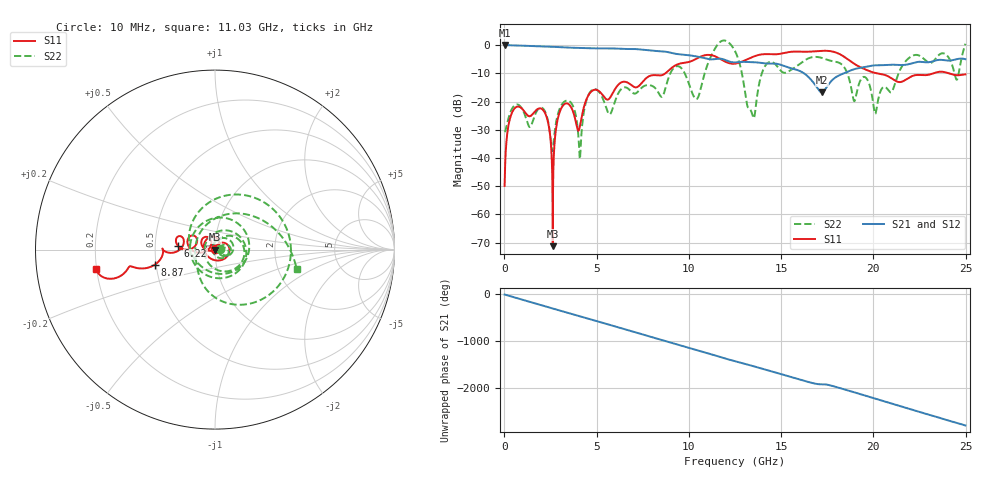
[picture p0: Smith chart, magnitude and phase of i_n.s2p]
!Keysight Technologies,N5245B,MY57181346,A.12.70.07
!Automatic Fixture Removal (AFR)
!Date: Wednesday, November 07, 2018 11:53:51 AM
!S2P File: Measurements: S11,S21,S12,S22:
# MHz S  RI  R 50
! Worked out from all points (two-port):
!   2499 points, 10 MHz to 24.99 GHz, reference 50 ohm
!   highest |S21| = 0.00 dB at 10 MHz (marker M1); lowest = -16.8 dB at 17.21 GHz (marker M2)
!   |S21| within 3 dB of the highest: start of sweep to 9.215 GHz
!   lowest |S11| = -71.3 dB at 2.62 GHz (marker M3), VSWR 1.00, Z = 50 - j0.0251 ohm
!   |S11| at or under -10 dB: start of sweep to 8.728 GHz; 20.19 GHz to 23.26 GHz (3.073 GHz wide, 14.1 % of centre); 24.08 GHz to end of sweep
!   |S22| runs from -40.4 to 1.6 dB; largest |S21 - S12| = 1.4e-15
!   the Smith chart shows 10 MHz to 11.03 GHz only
!   S11 on the Smith chart (normalised r, x): 10 MHz: 1.01, +0.00; 6.22 GHz: 0.66, +0.03; 8.87 GHz: 0.49, -0.09; 11.03 GHz: 0.20, -0.08
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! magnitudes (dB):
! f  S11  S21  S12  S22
! 10 MHz  -49.9  0.0  0.0  -30.8
! 710 MHz  -21.8  -0.2  -0.2  -21.1
! 2.15 GHz  -23.5  -0.5  -0.5  -23.0
! 2.62 GHz  -71.3  -0.6  -0.6  -37.0
! 3.14 GHz  -21.7  -0.8  -0.8  -20.8
! 4.18 GHz  -25.7  -1.0  -1.0  -31.0
! 4.69 GHz  -16.6  -1.1  -1.1  -16.3
! 6.22 GHz  -13.7  -1.3  -1.3  -16.5
! 8.34 GHz  -10.8  -2.1  -2.1  -16.8
! 8.87 GHz  -9.2  -2.5  -2.5  -12.1
! 10.42 GHz  -4.8  -4.0  -4.0  -19.1
! 11.03 GHz  -3.5  -4.9  -4.9  -6.6
! 12.5 GHz  -6.6  -6.1  -6.1  -2.1
! 13.48 GHz  -4.1  -6.1  -6.1  -25.5
! 14.24 GHz  -3.2  -6.5  -6.5  -6.5
! 16.67 GHz  -2.3  -12.6  -12.6  -4.3
! 17.21 GHz  -2.0  -16.8  -16.8  -4.6
! 20.1 GHz  -9.9  -7.2  -7.2  -24.4
! 20.83 GHz  -11.2  -7.0  -7.0  -16.2
! 22.24 GHz  -10.7  -6.2  -6.2  -3.5
! 24.53 GHz  -10.7  -5.0  -5.0  -12.3
! 24.99 GHz  -10.4  -5.0  -5.0  0.5
